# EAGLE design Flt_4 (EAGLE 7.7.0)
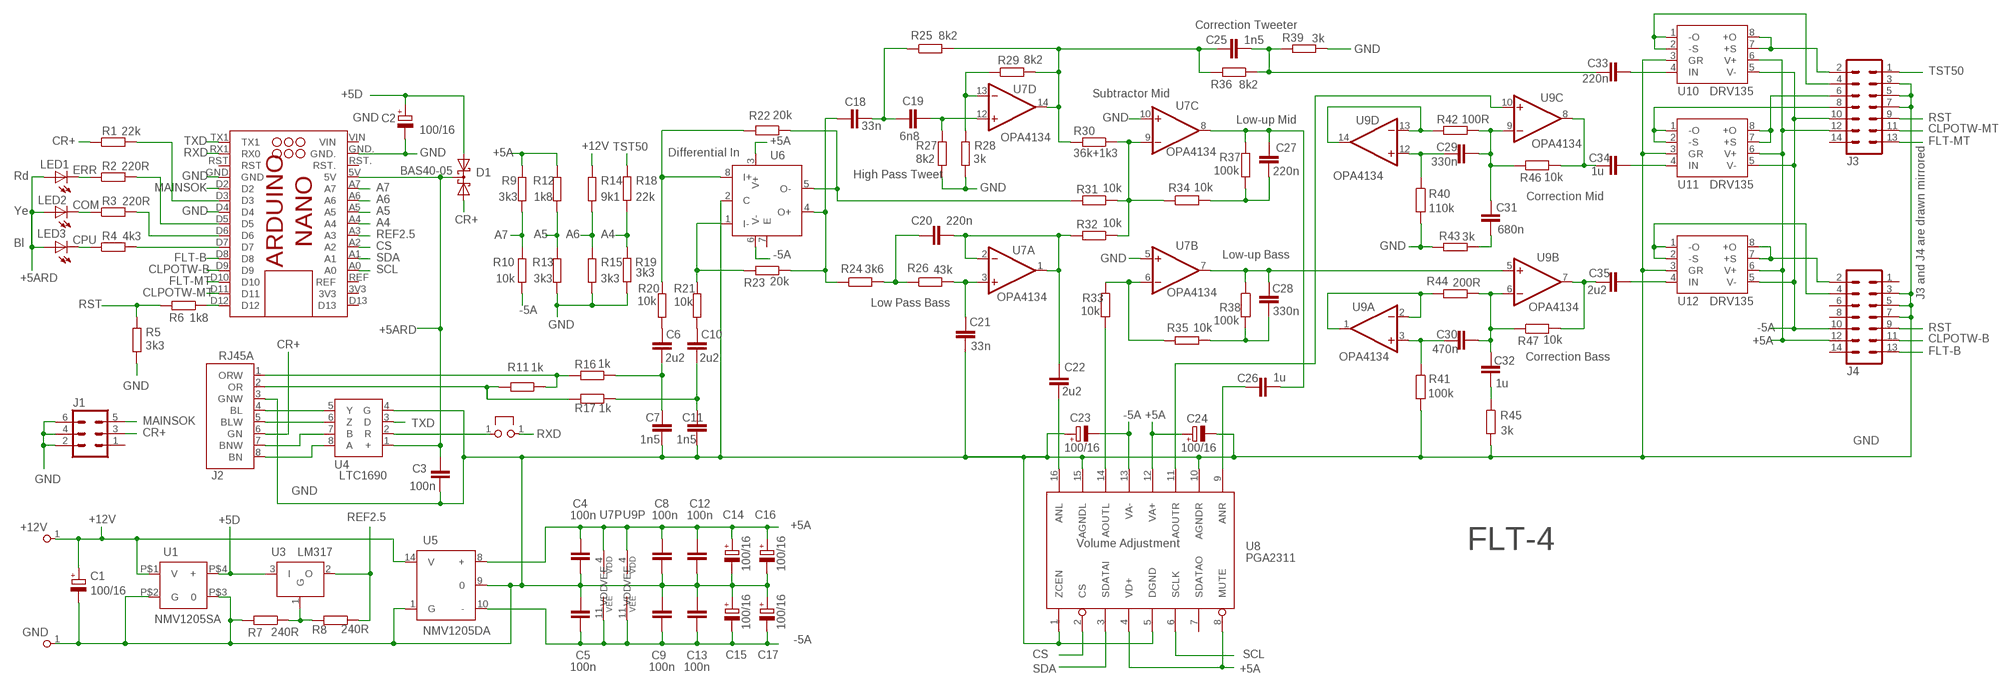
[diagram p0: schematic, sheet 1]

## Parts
+12V  PINHDR-1X1  [HDR1X1]
C1  100/16  CPOL-EUE2.5-7  [E2,5-7]
C2  100/16  CPOL-EUE2.5-7  [E2,5-7]
C3  100n  C-EU050-024X044  [C050-024X044]
C4  100n  C-EU050-024X044  [C050-024X044]
C5  100n  C-EU050-024X044  [C050-024X044]
C6  2u2  C-EU050-075X075  [C050-075X075]
C7  1n5  C-EU075-032X103  [C075-032X103]
C8  100n  C-EU050-024X044  [C050-024X044]
C9  100n  C-EU050-024X044  [C050-024X044]
C10  2u2  C-EU050-075X075  [C050-075X075]
C11  1n5  C-EU075-032X103  [C075-032X103]
C12  100n  C-EU050-024X044  [C050-024X044]
C13  100n  C-EU050-024X044  [C050-024X044]
C14  100/16  CPOL-EUE2.5-7  [E2,5-7]
C15  100/16  CPOL-EUE2.5-7  [E2,5-7]
C16  100/16  CPOL-EUE2.5-7  [E2,5-7]
C17  100/16  CPOL-EUE2.5-7  [E2,5-7]
C18  33n  C-EU075-032X103  [C075-032X103]
C19  6n8  C-EU075-032X103  [C075-032X103]
C20  220n  C-EU050-030X075  [C050-030X075]
C21  33n  C-EU075-032X103  [C075-032X103]
C22  2u2  C-EU050-075X075  [C050-075X075]
C23  100/16  CPOL-EUE2.5-7  [E2,5-7]
C24  100/16  CPOL-EUE2.5-7  [E2,5-7]
C25  1n5  C-EU050-045X075  [C050-045X075]
C26  1u  C-EU050-050X075  [C050-050X075]
C27  220n  C-EU050-030X075  [C050-030X075]
C28  330n  C-EU050-035X075  [C050-035X075]
C29  330n  C-EU050-035X075  [C050-035X075]
C30  470n  C-EU050-035X075  [C050-035X075]
C31  680n  C-EU050-045X075  [C050-045X075]
C32  1u  C-EU050-050X075  [C050-050X075]
C33  220n  C-EU050-030X075  [C050-030X075]
C34  1u  C-EU050-050X075  [C050-050X075]
C35  2u2  C-EU050-075X075  [C050-075X075]
D1  BAS40-05  DDIODE_ACA  [SOT23]
GND  PINHDR-1X1  [HDR1X1]
J1  PINHD-3X2  [MA03-2]
J2  RJ45A  [1XRJ45_MM_JACK]
J3  PINHD-7X2  [MA07-2]
J4  PINHD-7X2  [MA07-2]
LED1  Rd  LED3MM  [LED3MM]
LED2  Ye  LED3MM  [LED3MM]
LED3  Bl  LED3MM  [LED3MM]
R1  22k  R-EU_0207/10  [0207/10]
R2  220R  R-EU_0207/10  [0207/10]
R3  220R  R-EU_0207/10  [0207/10]
R4  4k3  R-EU_0207/10  [0207/10]
R5  3k3  R-EU_0207/10  [0207/10]
R6  1k8  R-EU_0207/10  [0207/10]
R7  240R  R-EU_0207/10  [0207/10]
R8  240R  R-EU_0207/10  [0207/10]
R9  3k3  R-EU_0207/10  [0207/10]
R10  10k  R-EU_0207/10  [0207/10]
R11  1k  R-EU_0207/10  [0207/10]
R12  1k8  R-EU_0207/10  [0207/10]
R13  3k3  R-EU_0207/10  [0207/10]
R14  9k1  R-EU_0207/10  [0207/10]
R15  3k3  R-EU_0207/10  [0207/10]
R16  1k  R-EU_0207/10  [0207/10]
R17  1k  R-EU_0207/10  [0207/10]
R18  22k  R-EU_0207/10  [0207/10]
R19  3k3  R-EU_0207/10  [0207/10]
R20  10k  R-EU_0207/10  [0207/10]
R21  10k  R-EU_0207/10  [0207/10]
R22  20k  R-EU_0207/10  [0207/10]
R23  20k  R-EU_0207/10  [0207/10]
R24  3k6  R-EU_0207/10  [0207/10]
R25  8k2  R-EU_0207/10  [0207/10]
R26  43k  R-EU_0207/10  [0207/10]
R27  8k2  R-EU_0207/10  [0207/10]
R28  3k  R-EU_0207/10  [0207/10]
R29  8k2  R-EU_0207/10  [0207/10]
R30  36k+1k3  R-EU_0207/10  [0207/10]
R31  10k  R-EU_0207/10  [0207/10]
R32  10k  R-EU_0207/10  [0207/10]
R33  10k  R-EU_0207/10  [0207/10]
R34  10k  R-EU_0207/10  [0207/10]
R35  10k  R-EU_0207/10  [0207/10]
R36  8k2  R-EU_0207/10  [0207/10]
R37  100k  R-EU_0207/10  [0207/10]
R38  100k  R-EU_0207/10  [0207/10]
R39  3k  R-EU_0207/10  [0207/10]
R40  110k  R-EU_0207/10  [0207/10]
R41  100k  R-EU_0207/10  [0207/10]
R42  100R  R-EU_0207/10  [0207/10]
R43  3k  R-EU_0207/10  [0207/10]
R44  200R  R-EU_0207/10  [0207/10]
R45  3k  R-EU_0207/10  [0207/10]
R46  10k  R-EU_0207/10  [0207/10]
R47  10k  R-EU_0207/10  [0207/10]
RXD  PINHDR-1X1  [HDR1X1]
RXD.  PINHDR-1X1  [HDR1X1]
U1  NMV1205SA  [NMV1205SA]
U2  ARDUINO_NANO_NOICSP  [ARDUINO_NANO_NOICSP]
U3  LM317  [TO92]
U4  LTC1690  [SO08]
U5  NMV1205DA  [NMV1205DA]
U6  OPA1632  [SO08]
U7  OPA4134  LM124  [SO14]
U8  PGA2311  PGA2311U  [SO16-1]
U9  OPA4134  LM124  [SO14]
U10  DRV135  [SO08]
U11  DRV135  [SO08]
U12  DRV135  [SO08]

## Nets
+5A: C4.2 C8.2 C12.2 C14.+ C16.+ C24.+ J3.12 J4.12 R9.1 R12.1 U5.8(+) U6.3(V+) U7.4(P:VDD) U8.4(VD+) U8.8(MUTE) U8.12(VA+) U9.4(P:VDD) U10.6(V+) U11.6(V+) U12.6(V+)
+5ARD: C3.2 D1.3(C) LED1.A LED2.A LED3.A U2.5V U4.1(+)
+5D: C2.+ D1.2(A2) U1.P$4(+) U3.3(I)
+12V: +12V.1 C1.+ R14.1 U1.P$1(V) U5.14(V)
-5A: C5.1 C9.1 C13.1 C15.- C17.- C23.- J3.10 J4.10 R10.2 U5.10(-) U6.6(V-) U7.11(P:VEE) U8.13(VA-) U9.11(P:VEE) U10.5(V-) U11.5(V-) U12.5(V-)
A4: R18.1 R19.2 U2.A4
A5: R12.2 R13.1 U2.A5
A6: R14.2 R15.1 U2.A6
A7: R9.2 R10.1 U2.A7
CLPOTW-B: J4.11 U2.D9
CLPOTW-MT: J3.11 U2.D11
COM: R3.2 U2.D6
CPU: R4.2 U2.D7
CR+: D1.1(A1) J1.3 J2.6(GN) R1.1
CS: U2.A2 U8.2(CS)
ERR: R2.2 U2.D5
FLT-B: J4.13 U2.D8
FLT-MT: J3.13 U2.D10
GND: C2.- C3.1 C4.1 C5.2 C7.1 C8.1 C9.2 C11.1 C12.1 C13.2 C14.- C15.+ C16.- C17.+ C21.1 C23.+ C24.- GND.1 J1.2 J1.4 J1.6 J2.3(GNW) J3.3 J3.5 J3.7 J4.3 J4.5 J4.7 R5.1 R7.2 R13.2 R15.2 R19.1 R27.1 R28.1 R39.2 R40.2 R41.2 R43.2 R45.2 U1.P$2(G) U1.P$3 U2.D4 U2.GND U2.GND. U4.4(G) U5.1(G) U5.9 U6.2(C) U7.5(B:+IN) U7.10(C:+IN) U8.1(ZCEN) U8.5(DGND) U8.10(AGNDR) U8.15(AGNDL) U10.3(GR) U11.3(GR) U12.3(GR)
MAINSOK: J1.5 U2.D2
MI: C26.2 C27.2 R37.2 U7.8(C:OUT)
MO: U8.11(AOUTR) U9.10(C:+IN)
N$1: C30.2 C32.2 R44.1 R47.1 U9.6(B:-IN)
N$2: R44.2 U9.1(A:OUT) U9.2(A:-IN)
N$3: R6.1 U2.D12
N$4: R30.1 R31.1 R32.1 R34.1 U7.9(C:-IN)
N$5: C28.2 R38.1 U7.7(B:OUT) U9.5(B:+IN)
N$6: C30.1 R41.1 U9.3(A:+IN)
N$7: C18.1 R23.1 R24.1 U6.4(O+)
N$8: C32.1 R45.1
N$9: J3.8 U11.1(-O) U11.2(-S)
N$10: R20.1 R22.2 U6.8(I+)
N$11: C28.1 R35.1 R38.2
N$12: C27.1 R34.2 R37.1
N$13: J3.2 U10.7(+S) U10.8(+O)
N$14: C20.1 R24.2 R26.1
N$15: C29.2 C31.2 R42.1 R46.1 U9.9(C:-IN)
N$16: C35.1 R47.2 U9.7(B:OUT)
N$17: C34.1 R46.2 U9.8(C:OUT)
N$18: C25.2 C33.1 R36.1 R39.1
N$19: C18.2 C19.1 R25.1
N$20: C6.2 R20.2
N$21: R42.2 U9.13(D:-IN) U9.14(D:OUT)
N$22: R21.1 R23.2 U6.1(I-)
N$23: C29.1 R40.1 U9.12(D:+IN)
N$24: R28.2 R29.1 U7.13(D:-IN)
N$25: R33.1 R35.2 U7.6(B:-IN)
N$26: C10.2 R21.2
N$27: C20.2 C22.1 R32.2 U7.1(A:OUT) U7.2(A:-IN)
N$28: J3.6 U11.7(+S) U11.8(+O)
N$30: R33.2 U8.14(AOUTL)
N$31: R22.1 R31.2 U6.5(O-)
N$32: R1.2 U2.D3
N$33: R7.1 R8.2 U3.1(G)
N$34: C31.1 R43.1
N$35: J3.4 U10.1(-O) U10.2(-S)
N$36: C22.2 U8.16(ANL)
N$37: C26.1 U8.9(ANR)
N$38: C6.1 C7.2 R16.1
N$39: C10.1 C11.2 R17.1
N$40: C19.2 R27.2 U7.12(D:+IN)
N$41: C33.2 U10.4(IN)
N$42: C34.2 U11.4(IN)
N$43: C21.2 R26.2 U7.3(A:+IN)
N$44: J2.8(BN) U4.8(A)
N$45: J2.7(BNW) U4.7(B)
N$46: C35.2 U12.4(IN)
N$47: J4.2 U12.7(+S) U12.8(+O)
N$48: J2.5(BLW) U4.6(Z)
N$49: C1.-
N$56: J2.4(BL) U4.5(Y)
N$69: J4.4 U12.1(-O) U12.2(-S)
N$73: LED1.K(C) R2.1
N$74: LED2.K(C) R3.1
N$75: LED3.K(C) R4.1
NEGIN: J2.1(ORW) R11.1 R16.2
POSIN: J2.2(OR) R11.2 R17.2
REF2.5: R8.1 U2.A3 U3.2(O)
RST: J3.9 J4.9 R5.2 R6.2
RXD: RXD.1 U2.RX1(RX0)
RXD.: RXD..1 U4.2(R)
SCL: U2.A0 U8.6(SCLK)
SDA: U2.A1 U8.3(SDATAI)
TST50: J3.1 R18.2
TW: C25.1 R25.2 R29.2 R30.2 R36.2 U7.14(D:OUT)
TXD: U2.TX1 U4.3(D)
Unconnected: J1.1 J3.14 J4.1 J4.6 J4.8 J4.14 U2.3V3 U2.D13 U2.REF U2.RST U2.RST. U2.VIN U6.7(E) U8.7(SDATAO)

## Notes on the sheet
- Correction Tweeter
- Subtractor Mid
- Low-up Mid
- Differential In
- High Pass Tweet
- Correction Mid
- Low-up Bass
- J3 and J4 are drawn mirrored
- Low Pass Bass
- Correction Bass
- Volume Adjustment | FLT-4

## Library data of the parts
+12V GND RXD RXD. = Header:PINHDR-1X1
C1 C2 C14-C17 C23 C24 = 0A-Passive:CPOL-EU: POLARIZED CAPACITOR, European symbol
C3-C13 C18-C22 C25-C35 = AJANLIB:C-EU: CAPACITOR, European symbol
D1 = DiodeRect:DDIODE_ACA: Silicon Schottky Diodes General-purpose diode for high-speed switching
J1 = Header:PINHD-3X2: PIN HEADER
J2 = Connector:RJ45A
J3 J4 = Header:PINHD-7X2: PIN HEADER
LED1-LED3 = Opto:LED: LED
R1-R6 R18 R19 = Passive:R-EU_: RESISTOR, European symbol
R7-R17 R20-R47 = AJANLIB:R-EU_: RESISTOR, European symbol
U1 = Regulator:NMV1205SA
U2 = arduinos:ARDUINO_NANO_NOICSP
U3 = Regulator:LM317
U4 = IC_Interface:LTC1690
U5 = Regulator:NMV1205DA
U6 = IC_Lin:OPA1632
U7 U9 = IC_Lin:LM124: Quad Op Amp
U8 = AJANLIB:PGA2311: Stereo Volume Control
U10-U12 = IC_Lin:DRV135

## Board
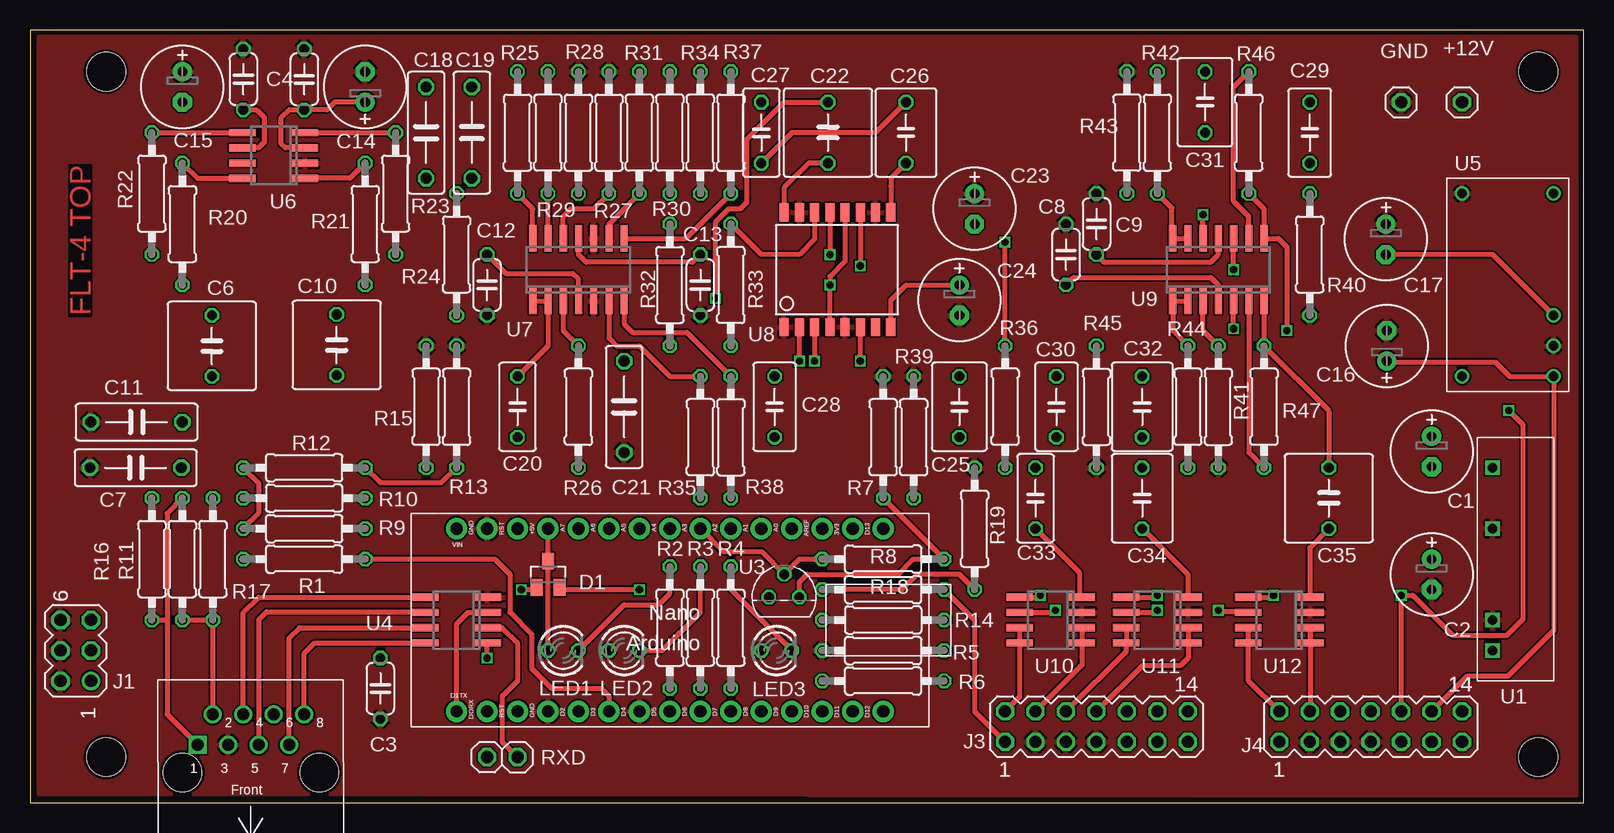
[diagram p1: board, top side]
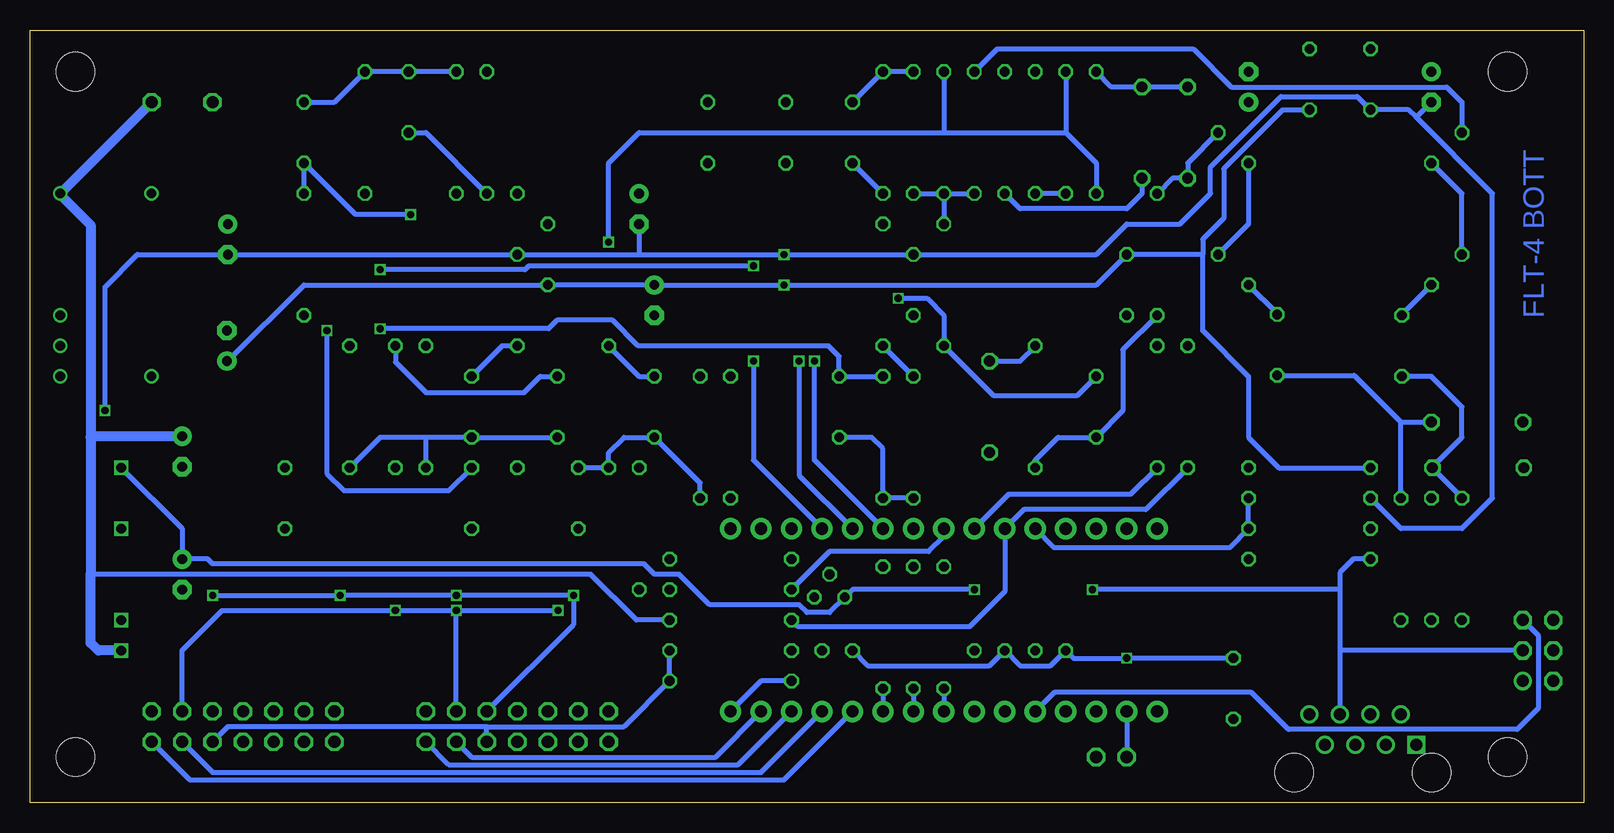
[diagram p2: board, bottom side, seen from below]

Size 129.52 x 64.44 mm. Coordinates in mm from the lower left corner, seen from the top.
Outline: 0,0 129.52,0 129.52,64.44 0,64.44 0,0
Copper layers (1*16): Top 0.018mm / dielectric 1.55mm / Bottom 0.018mm
Design rules "eC_2Layer_PClass6_BaseCopperO18_eCDefault *": minimum track width 0.15mm, minimum drill 0.35mm, track to track 0.15mm, track to pad 0.15mm, pad to pad 0.15mm, via to via 0.15mm, smd to smd 0mil, copper to edge 0.25mm, drill to drill 0.35mm, minimum pad ring 0.175mm, minimum via ring 0.125mm, stop-mask expansion 0mil, vias tented up to drill 0.45mm, thermal gap 0.2mm
Holes 3.2 mm at 6.35,3.81 125.73,3.81 125.73,60.96 6.35,60.96

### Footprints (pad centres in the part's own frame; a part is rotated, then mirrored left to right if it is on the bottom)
HDR1X1 = drill 1.016 octagon: 1 0,0
E2,5-7 = drill 0.813 pad 1.6: + -1.27,0 | drill 0.813 pad 1.6 octagon: - 1.27,0
C050-024X044 = drill 0.813 octagon: 1 -2.54,0; 2 2.54,0
C050-075X075 = drill 0.813 octagon: 1 -2.54,0; 2 2.54,0
C075-032X103 = drill 0.914 octagon: 1 -3.81,0; 2 3.81,0
C050-030X075 = drill 0.813 octagon: 1 -2.54,0; 2 2.54,0
C050-045X075 = drill 0.813 octagon: 1 -2.54,0; 2 2.54,0
C050-050X075 = drill 0.813 octagon: 1 -2.54,0; 2 2.54,0
C050-035X075 = drill 0.813 octagon: 1 -2.54,0; 2 2.54,0
SOT23 = smd 1 x 1.4: 1 -0.95,-1.1; 2 0.95,-1.1; 3 0,1.1
MA03-2 = drill 1.016: 1 -2.54,-1.27 | drill 1.016 octagon: 2 -2.54,1.27; 3 0,-1.27; 4 0,1.27; 5 2.54,-1.27; 6 2.54,1.27
1XRJ45_MM_JACK = drill 1 square: 1 4.445,-2.286 | drill 1: 2 3.175,-4.826; 3 1.905,-2.286; 4 0.635,-4.826; 5 -0.635,-2.286; 6 -1.905,-4.826; 7 -3.175,-2.286; 8 -4.445,-4.826 | hole 3.2: -5.715,0; 5.715,0
MA07-2 = drill 1.016 octagon: 1 -7.62,-1.27; 2 -7.62,1.27; 3 -5.08,-1.27; 4 -5.08,1.27; 5 -2.54,-1.27; 6 -2.54,1.27; 7 0,-1.27; 8 0,1.27; 9 2.54,-1.27; 10 2.54,1.27; 11 5.08,-1.27; 12 5.08,1.27; 13 7.62,-1.27; 14 7.62,1.27
LED3MM = drill 0.813 octagon: A -1.27,0; K 1.27,0
0207/10 = drill 0.813 octagon: 1 -5.08,0; 2 5.08,0
NMV1205SA = drill 0.8 square: P$1 -7.62,0; P$2 -5.08,0; P$3 2.54,0; P$4 7.62,0
ARDUINO_NANO_NOICSP = drill 1.016 pad 1.778: 3V3 6.35,1.27; 5V 31.75,1.27; A0 11.43,1.27; A1 13.97,1.27; A2 16.51,1.27; A3 19.05,1.27; A4 21.59,1.27; A5 24.13,1.27; A6 26.67,1.27; A7 29.21,1.27; D2 29.21,16.51; D3 26.67,16.51; D4 24.13,16.51; D5 21.59,16.51; D6 19.05,16.51; D7 16.51,16.51; D8 13.97,16.51; D9 11.43,16.51; D10 8.89,16.51; D11 6.35,16.51; D12 3.81,16.51; D13 3.81,1.27; GND 31.75,16.51; GND. 36.83,1.27; REF 8.89,1.27; RST 34.29,16.51; RST. 34.29,1.27; RX1 36.83,16.51; TX1 39.37,16.51; VIN 39.37,1.27
TO92 = drill 0.813 octagon: 1 1.27,0; 2 0,1.905; 3 -1.27,0
SO08 = smd 0.6 x 2.2: 1 -1.905,-2.6; 2 -0.635,-2.6; 3 0.635,-2.6; 4 1.905,-2.6; 5 1.905,2.6; 6 0.635,2.6; 7 -0.635,2.6; 8 -1.905,2.6
NMV1205DA = drill 0.8: 1 -7.62,-2.54; 7 7.62,-2.54; 8 7.62,5.08; 9 5.08,5.08; 10 2.54,5.08; 14 -7.62,5.08
SO14 = smd 0.6 x 2.2: 1 -3.81,-2.6; 2 -2.54,-2.6; 3 -1.27,-2.6; 4 0,-2.6; 5 1.27,-2.6; 6 2.54,-2.6; 7 3.81,-2.6; 8 3.81,2.6; 9 2.54,2.6; 10 1.27,2.6; 11 0,2.6; 12 -1.27,2.6; 13 -2.54,2.6; 14 -3.81,2.6
SO16-1 = smd 0.762 x 1.524: 1 -4.445,-4.775; 2 -3.175,-4.775; 3 -1.905,-4.775; 4 -0.635,-4.775; 5 0.635,-4.775; 6 1.905,-4.775; 7 3.175,-4.775; 8 4.445,-4.775; 9 4.445,4.775; 10 3.175,4.775; 11 1.905,4.775; 12 0.635,4.775; 13 -0.635,4.775; 14 -1.905,4.775; 15 -3.175,4.775; 16 -4.445,4.775

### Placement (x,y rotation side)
+12V  119.38,58.42 0 top
C1  116.84,29.29 270 top
C2  116.84,19.05 270 top
C3  29.21,9.53 90 top
C4  22.86,60.32 270 top
C5  17.78,60.32 90 top
C6  15.16,38.1 90 top
C7  8.81,27.94 0 top
C8  86.36,45.72 270 top
C9  88.9,48.26 90 top
C10  25.56,38.18 90 top
C11  8.89,31.75 0 top
C12  38.1,43.18 90 top
C13  55.88,43.18 270 top
C14  27.94,59.69 90 top
C15  12.7,59.69 270 top
C16  113.11,38.1 90 top
C17  113.03,46.99 270 top
C18  33.02,55.88 90 top
C19  36.83,55.88 270 top
C20  40.64,33.02 90 top
C21  49.53,33.02 90 top
C22  66.52,55.88 270 top
C23  78.74,49.53 270 top
C24  77.47,41.91 270 top
C25  77.47,33.02 270 top
C26  73.03,55.88 90 top
C27  60.96,55.88 270 top
C28  62.07,33.02 90 top
C29  106.68,55.88 90 top
C30  85.57,33.02 270 top
C31  97.95,58.42 90 top
C32  92.71,33.02 270 top
C33  83.82,25.4 270 top
C34  92.71,25.4 270 top
C35  108.27,25.4 270 top
D1  43.18,19.05 0 top
GND  114.3,58.42 0 top
J1  3.81,12.7 90 top
J2  18.41,2.54 180 top
J3  88.9,6.35 0 top
J4  111.76,6.35 0 top
LED1  44.45,12.7 0 top
LED2  49.53,12.7 0 top
LED3  62.23,12.7 0 top
R1  22.86,20.32 0 top
R2  53.34,14.61 270 top
R3  55.88,14.61 270 top
R4  58.42,14.61 270 top
R5  71.12,12.7 0 top
R6  71.12,10.16 0 top
R7  71.12,30.48 90 top
R8  71.12,20.32 0 top
R9  22.86,22.86 0 top
R10  22.86,25.4 180 top
R11  12.7,20.32 270 top
R12  22.86,27.94 0 top
R13  35.56,33.02 90 top
R14  71.12,15.24 180 top
R15  33.02,33.02 90 top
R16  10.16,20.32 270 top
R17  15.24,20.32 270 top
R18  71.12,17.78 0 top
R19  78.74,22.86 270 top
R20  12.7,48.26 270 top
R21  27.94,48.26 270 top
R22  10.16,50.8 270 top
R23  30.48,50.8 270 top
R24  35.56,45.72 270 top
R25  40.64,55.88 270 top
R26  45.72,33.02 90 top
R27  48.26,55.88 270 top
R28  45.72,55.88 270 top
R29  43.18,55.88 90 top
R30  53.34,55.88 90 top
R31  50.8,55.88 90 top
R32  53.34,43.18 270 top
R33  58.42,43.18 90 top
R34  55.88,55.88 90 top
R35  55.88,30.48 90 top
R36  81.28,33.02 90 top
R37  58.42,55.88 270 top
R38  58.42,30.48 270 top
R39  73.66,30.48 90 top
R40  106.68,45.72 270 top
R41  99.06,33.02 270 top
R42  93.98,55.88 270 top
R43  91.44,55.88 90 top
R44  96.52,33.02 90 top
R45  88.9,33.02 270 top
R46  101.6,55.88 270 top
R47  102.87,33.02 90 top
RXD  38.1,3.81 90 top
RXD.  40.64,3.81 0 top
U1  121.92,20.32 90 top
U2  74.93,24.13 180 top
U3  62.87,17.14 0 top
U4  35.56,15.24 90 top
U5  121.92,43.18 270 top
U6  20.32,53.98 90 top
U7  45.72,44.45 0 top
U8  67.31,44.45 0 top
U9  99.06,44.45 0 top
U10  85.09,15.24 90 top
U11  93.98,15.24 90 top
U12  104.14,15.24 90 top

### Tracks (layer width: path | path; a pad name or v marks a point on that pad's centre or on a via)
+5A  (via drill 0.6)
  Top 0.406: U6.3 21.27,54.61 20.95,54.93 20.95,57.15 21.59,57.78 C4.2 24.77,57.78 25.4,58.42 C14.+ | C8.2 87,43.81 98.43,43.81 99.06,43.18 U9.4 | C12.2 39.69,44.13 45.24,44.13 45.72,43.66 U7.4 | U8.8 71.76,41.91 73.03,43.18 C24.+ | U8.4 v66.68,43.18 66.68,43.89 67.95,45.16 U8.12 | R12.1 19.05,26.67 19.05,24.13 R9.1 | v99.06,16.03 99.06,15.95 99.06,15.96 101.46,15.96 101.46,15.95 U12.6 | C16.+ 113.19,36.75 122.16,36.75 123.35,35.56 U5.8 127,14.37 123.19,10.56 119.78,10.56 J4.12 | U11.6 93.82,15.88 v93.98,16.03 | U10.6 85.33,15.88 v85.49,16.03
  Bottom 0.406: C4.2 25.08,57.78 30,52.86 30,48.74 31.75,46.99 31.75,45.72 | 31.75,45.72 31.75,39.37 27.94,35.56 27.94,30.48 25.4,27.94 R12.1 | 31.75,45.72 C12.2 40.64,43.18 v66.68,43.18 C24.+ C8.2 106.68,43.18 113.03,36.83 C16.+ | J4.12 116.84,12.7 113.51,16.03 v99.06,16.03 v93.98,16.03 | v93.98,16.03 v85.49,16.03 | J3.12 v93.98,16.03
+5ARD  (via drill 0.6)
  Top 0.406: D1.3 U2.5V LED1.A | v38.1,12.07 38.1,13.27 U4.1
  Bottom 0.406: C3.2 v38.1,12.07 42.55,12.07 LED1.A 44.45,11.43 46.99,11.43 LED2.A 49.53,11.43 59.69,11.43 LED3.A
+5D  (via drill 0.6)
  Top 0.406: D1.2 44.3,17.78 v50.8,17.78
  Bottom 0.406: U1.P$4 116.84,22.86 C2.+ 114.7,20.32 114.3,19.92 78.34,19.92 77.47,19.05 75.41,19.05 72.87,16.51 65.41,16.51 64.77,15.88 62.87,15.88 U3.3 60.96,17.78 v50.8,17.78
+12V
  Bottom 0.406: 124.46,19.05 82.79,19.05 78.98,15.24 R14.1 | 124.38,30.56 124.46,30.48
  Bottom 0.813: U1.P$1 123.83,12.7 124.46,13.34 124.46,19.05 124.46,30.48 124.46,48.18 127,50.72 U5.14 +12V.1 | C1.+ 124.38,30.56
-5A  (via drill 0.6)
  Top 0.406: C5.1 18.89,57.78 19.53,57.15 19.53,55.09 19.05,54.61 U6.6 | C13.1 55.24,45.09 46.35,45.09 45.72,45.72 U7.11 | C9.1 89.54,45.09 98.43,45.09 99.06,45.72 U9.11 | U8.13 v66.68,45.72 | J4.10 v114.3,17.3 115.25,17.3 118.59,13.97 123.11,13.97 124.46,15.32 124.46,31.51 v123.27,32.7 | U5.10 121.92,45.72 C17.- | U12.5 103.51,17.14 v103.66,17.3 | U11.5 93.82,17.14 v93.98,17.3 | U10.5 84.06,17.14 v84.22,17.3
  Bottom 0.406: 13.97,57.15 7.62,50.8 7.62,25.4 10.16,22.86 15.24,22.86 R10.2 | 78.74,45.72 C9.1 C17.- 120.57,45.72 123.27,43.02 v123.27,32.7 | 78.74,45.72 v66.68,45.72 C13.1 40.64,45.72 38.1,48.26 33.66,48.26 31.11,50.8 31.11,53.02 25.24,58.9 18.89,58.9 C5.1 14.61,57.78 13.97,57.15 | C15.- 13.97,57.15 | C23.- 78.74,45.72 | v114.3,17.3 v103.66,17.3 v93.98,17.3 v84.22,17.3 84.22,14.84 J3.10
A4
  Top 0.406: R19.2 77.47,19.05 73.98,19.05 72.71,17.78 R18.1
  Bottom 0.406: R18.1 62.87,20.95 54.61,20.95 53.34,22.22 U2.A4
A5
  Top 0.406: R13.1 34.29,26.67 29.21,26.67 R12.2
  Bottom 0.406: R13.1 37.78,25.72 47.94,25.72 U2.A5
A6
  Bottom 0.406: R15.1 36.51,24.45 46.67,24.45 U2.A6 48.26,17.62 51.2,14.68 65.48,14.68 R14.2
A7
  Bottom 0.406: R10.1 R9.2 29.53,21.27 44.13,21.27 U2.A7
CLPOTW-B
  Bottom 0.406: U2.D9 68.58,2.54 114.3,2.54 J4.11
CLPOTW-MT
  Bottom 0.406: U2.D11 72.39,3.81 92.71,3.81 J3.11
COM
  Bottom 0.406: R3.2 U2.D6
CPU
  Bottom 0.406: R4.2 U2.D7
CR+  (via drill 0.6)
  Top 0.406: v40.96,17.78 42.06,17.78 D1.1
  Bottom 0.406: 20.32,17.78 v40.96,17.78 | 20.32,17.78 20.32,12.7 | 20.32,12.7 J2.6 | R1.1 19.21,20.32 20.32,19.21 20.32,17.78 | J1.3 20.32,12.7
CS  (via drill 0.6)
  Top 0.406: v64.14,36.83 U8.2
  Bottom 0.406: v64.14,36.83 64.14,28.57 U2.A2
ERR
  Bottom 0.406: R2.2 U2.D5
FLT-B
  Bottom 0.406: U2.D8 66.68,1.91 116.21,1.91 J4.13
FLT-MT
  Bottom 0.406: U2.D10 70.48,3.17 94.62,3.17 J3.13
GND
  pour Top: 0.71,0.79 128.91,0.64 128.91,63.82 0.71,63.82
MAINSOK
  Bottom 0.406: J1.5 3.81,13.97 3.81,7.86 5.56,6.11 24.61,6.11 27.7,9.21 44.13,9.21 U2.D2
MI
  Top 0.406: C26.2 70.48,55.88 63.5,55.88 C27.2 | U7.8 54.67,47.05 R37.2
  Bottom 0.406: R37.2 C27.2
MO  (via drill 0.6)
  Top 0.406: U8.11 v69.22,44.77 | v100.33,44.45 U9.10
  Bottom 0.406: v69.22,44.77 87.95,44.77 88.27,44.45 v100.33,44.45
N$1
  Top 0.406: U9.6 101.6,29.21 R47.1
  Bottom 0.406: 96.52,30.48 C32.2 C30.2 | 96.52,30.48 100.33,30.48 R47.1 | R44.1 96.52,30.48
N$2
  Top 0.406: U9.2 U9.1 95.25,39.37 R44.2
N$3
  Bottom 0.406: R6.1 68.58,10.16 U2.D12
N$4
  Top 0.406: U7.9 48.26,48.26 R31.1
  Bottom 0.406: R34.1 R30.1 | R30.1 R31.1 | R30.1 R32.1
N$5  (via drill 0.6)
  Top 0.406: U7.7 49.53,39.93 50.24,39.21 54.77,39.21 R38.1 | v100.33,39.53 U9.5
  Bottom 0.406: v100.33,39.53 86.28,39.53 85.57,40.24 80.96,40.24 78.82,38.1 62.94,38.1 62.07,37.23 C28.2 R38.1
N$6
  Top 0.406: R41.1 97.79,39.37 U9.3
  Bottom 0.406: R41.1 99.06,36.75 96.52,34.21 88.34,34.21 87,35.56 C30.1
N$7
  Top 0.406: U6.4 R23.1
  Bottom 0.406: R23.1 33.02,53.34 C18.1 34.29,52.07 R24.1
N$8
  Bottom 0.406: R45.1 90.17,38.1 C32.1
N$9
  Top 0.406: J3.8 92.71,11.43 95.89,11.43 96.52,12.07 96.58,12.12 U11.1 U11.2
N$10
  Top 0.406: R20.1 13.97,52.07 U6.8
  Bottom 0.406: R22.2 10.16,50.8 R20.1
N$11
  Bottom 0.406: R35.1 R38.2 58.42,29.53 59.37,30.48 C28.1
N$12
  Bottom 0.406: C27.1 R37.1 R34.2
N$13
  Top 0.406: J3.2 82.49,8.83 U10.8 U10.7
N$14
  Bottom 0.406: R24.2 38.42,37.78 38.42,32.7 C20.1 43.81,30.48 45.72,28.57 R26.1
N$15
  Top 0.406: U9.9 101.6,48.89 100.33,50.16 100.33,59.69 R46.1
  Bottom 0.406: C29.2 104.14,58.42 R46.1 C31.2 R42.1
N$16
  Top 0.406: U9.7 R47.2 108.27,32.7 C35.1
N$17  (via drill 0.6)
  Top 0.406: R46.2 102.87,49.53 U9.8 104.08,47.05 104.78,46.35 v104.78,39.37
  Bottom 0.406: v104.78,39.37 104.78,27.46 103.35,26.04 94.62,26.04 C34.1
N$18
  Bottom 0.406: R39.1 73.66,26.67 C25.2 80.01,30.48 81.28,29.21 R36.1 C33.1
N$19
  Bottom 0.406: C18.2 C19.1 39.37,59.69 R25.1
N$20
  Bottom 0.406: C6.2 15.16,40.72 R20.2
N$21
  Top 0.406: R42.2 95.19,49.59 95.19,46.99 U9.14 U9.13
N$22
  Top 0.406: R21.1 26.67,52.07 U6.1
  Bottom 0.406: R21.1 27.94,48.26 R23.2
N$23  (via drill 0.6)
  Top 0.406: U9.12 v97.79,49.05
  Bottom 0.406: R40.1 C29.1 102.39,49.05 v97.79,49.05
N$24
  Top 0.406: U7.13 R29.1
  Bottom 0.406: R29.1 R28.2
N$25
  Top 0.406: U7.6 48.26,38.73 48.89,38.1 50.8,38.1 53.34,35.56 R35.2
  Bottom 0.406: R35.2 R33.1
N$26
  Bottom 0.406: C10.2 25.56,40.8 R21.2
N$27  (via drill 0.6)
  Top 0.406: C20.2 43.18,38.1 U7.2 U7.1 | v57.15,42.07 57.15,48.42 58.26,49.53 59.21,49.53 59.77,50.09 59.77,55.32 62.87,58.42 C22.1
  Bottom 0.406: C20.2 42.23,33.97 49.21,33.97 R32.2 53.34,40.64 54.77,42.07 v57.15,42.07
N$28
  Top 0.406: J3.6 91.38,12.64 U11.8 U11.7
N$30
  Top 0.406: U8.14 65.41,46.99 64.14,45.72 60.96,45.72 R33.2
N$31
  Top 0.406: R22.1 U6.5
  Bottom 0.406: R31.2 48.89,62.87 32.54,62.87 29.37,59.69 11.43,59.69 10.16,58.42 R22.1
N$32
  Top 0.406: R1.2 38.73,20.32 40.01,19.05 40.01,15.88 41.83,14.05 41.83,11.19 43.5,9.53 47.62,9.53 48.26,8.89 U2.D3
N$33
  Top 0.406: U3.1 64.14,18.41 64.77,19.05 72.39,19.05 73.66,20.32 R8.2 R7.1
N$34
  Bottom 0.406: R43.1 96.52,55.88 C31.1
N$35
  Top 0.406: J3.4 87.69,11.49 U10.1 U10.2
N$36
  Top 0.406: C22.2 64.93,53.34 62.87,51.28 U8.16
N$37
  Top 0.406: C26.1 71.76,52.07 71.76,51.44 U8.9
N$38
  Bottom 0.406: R16.1 10.16,25.48 C7.2 12.62,28.02 10.16,30.48 10.16,33.02 12.7,35.56 C6.1
N$39
  Bottom 0.406: R17.1 15.24,31.75 | C10.1 19.13,35.64 15.24,31.75 | 15.24,31.75 C11.2
N$40
  Top 0.406: U7.12 44.45,48.89 45.09,49.53 46.99,49.53 R27.2
  Bottom 0.406: C19.2 36.83,50.8 38.1,49.53 46.99,49.53 R27.2
N$41
  Top 0.406: C33.2 87.47,19.21 87.47,17.36 U10.4
N$42
  Top 0.406: C34.2 96.52,19.05 96.52,17.2 U11.4
N$43
  Top 0.406: U7.3 44.45,39.37 R26.2
  Bottom 0.406: C21.2 46.99,36.83 R26.2
N$44
  Top 0.406: J2.8 22.86,12.46 23.73,13.34 U4.8
N$45
  Top 0.406: J2.7 21.59,13.73 22.46,14.61 U4.7
N$46
  Top 0.406: C35.2 106.68,21.27 106.68,17.2 U12.4
N$47
  Top 0.406: J4.2 101.54,10.22 U12.8 U12.7
N$48
  Top 0.406: J2.5 19.05,15.24 19.74,15.93 32.9,15.93 U4.6
N$56
  Top 0.406: J2.4 17.78,15.88 19.05,17.14 U4.5
N$69
  Top 0.406: U12.1 U12.2 106.68,14.61 106.68,13.39 U12.1 | U12.1 106.74,7.68 J4.4
N$73
  Top 0.406: LED1.K 49.53,16.51 52.39,16.51 53.34,17.46 R2.1
N$74
  Top 0.406: LED2.K 52.7,12.7 55.88,15.88 R3.1
N$75
  Top 0.406: LED3.K 58.42,17.78 R4.1
NEGIN
  Top 0.406: 11.43,15.24 11.43,24.13 R11.1 | R16.2 11.43,15.24 | 11.43,15.24 11.43,7.37 J2.1
POSIN
  Top 0.406: R11.2 R17.2 J2.2
REF2.5
  Top 0.406: U2.A3 57.78,20.95 60.96,20.95 U3.2 64.14,20.32 R8.1
RST
  Bottom 0.406: 91.44,6.35 80.01,6.35 R6.2 R5.2 | J3.9 91.44,6.35 | 91.44,6.35 113.03,6.35 J4.9
RXD
  Bottom 0.406: U2.RX1 RXD.1
RXD.
  Top 0.406: U4.2 39.37,14.61 40.64,13.34 40.64,10.16 39.37,8.89 39.37,5.08 RXD..1
SCL  (via drill 0.6)
  Top 0.406: v69.22,36.83 U8.6
  Bottom 0.406: v69.22,36.83 69.22,28.57 U2.A0
SDA  (via drill 0.6)
  Top 0.406: U8.3 v65.41,36.83
  Bottom 0.406: v65.41,36.83 65.41,27.3 U2.A1
TST50
  Top 0.406: J3.1 78.74,7.62 78.74,15.24 R18.2
TW  (via drill 0.6)
  Top 0.406: U7.14 41.91,49.53 R25.2 | R36.2 v81.28,46.75
  Bottom 0.406: v81.28,46.75 81.28,53.34 78.74,55.88 53.34,55.88 | R36.2 78.74,35.56 C25.1 | 53.34,55.88 43.18,55.88 | 43.18,55.88 40.64,53.34 R25.2 | R30.2 53.34,55.88 | R29.2 43.18,55.88
TXD
  Top 0.406: U2.TX1 35.56,14.92 36.51,15.88 U4.3

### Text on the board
Top: FLT-4 TOP
Bottom: FLT-4 BOTT
tNames: GND | RST | +5V | A7 | A6 | A5 | A4 | A3 | A2 | A1 | A0 | AREF | 3V3 | D13 | VIN | 6 | Nano | Arduino | 14 | D1TX | 2 | 4 | 6 | 8 | RST | GND | D2 | D3 | D4 | D5 | D6 | D7 | D8 | D9 | D10 | D11 | D12 | 1 | DORX | 1 | 3 | 5 | 7 | 1 | 1 | Front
